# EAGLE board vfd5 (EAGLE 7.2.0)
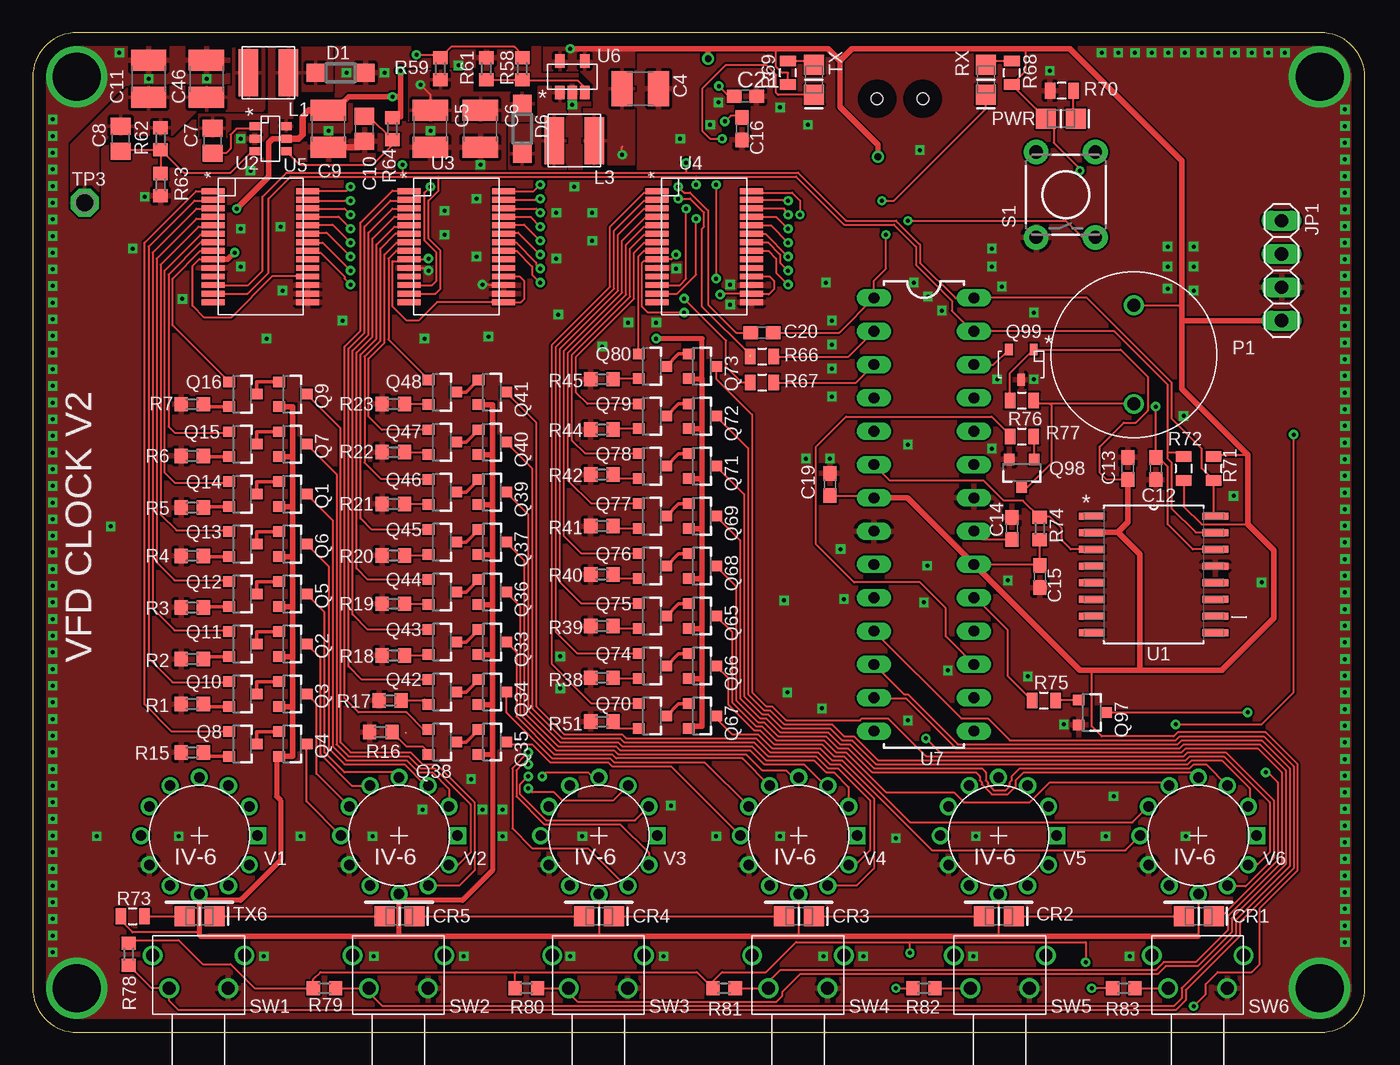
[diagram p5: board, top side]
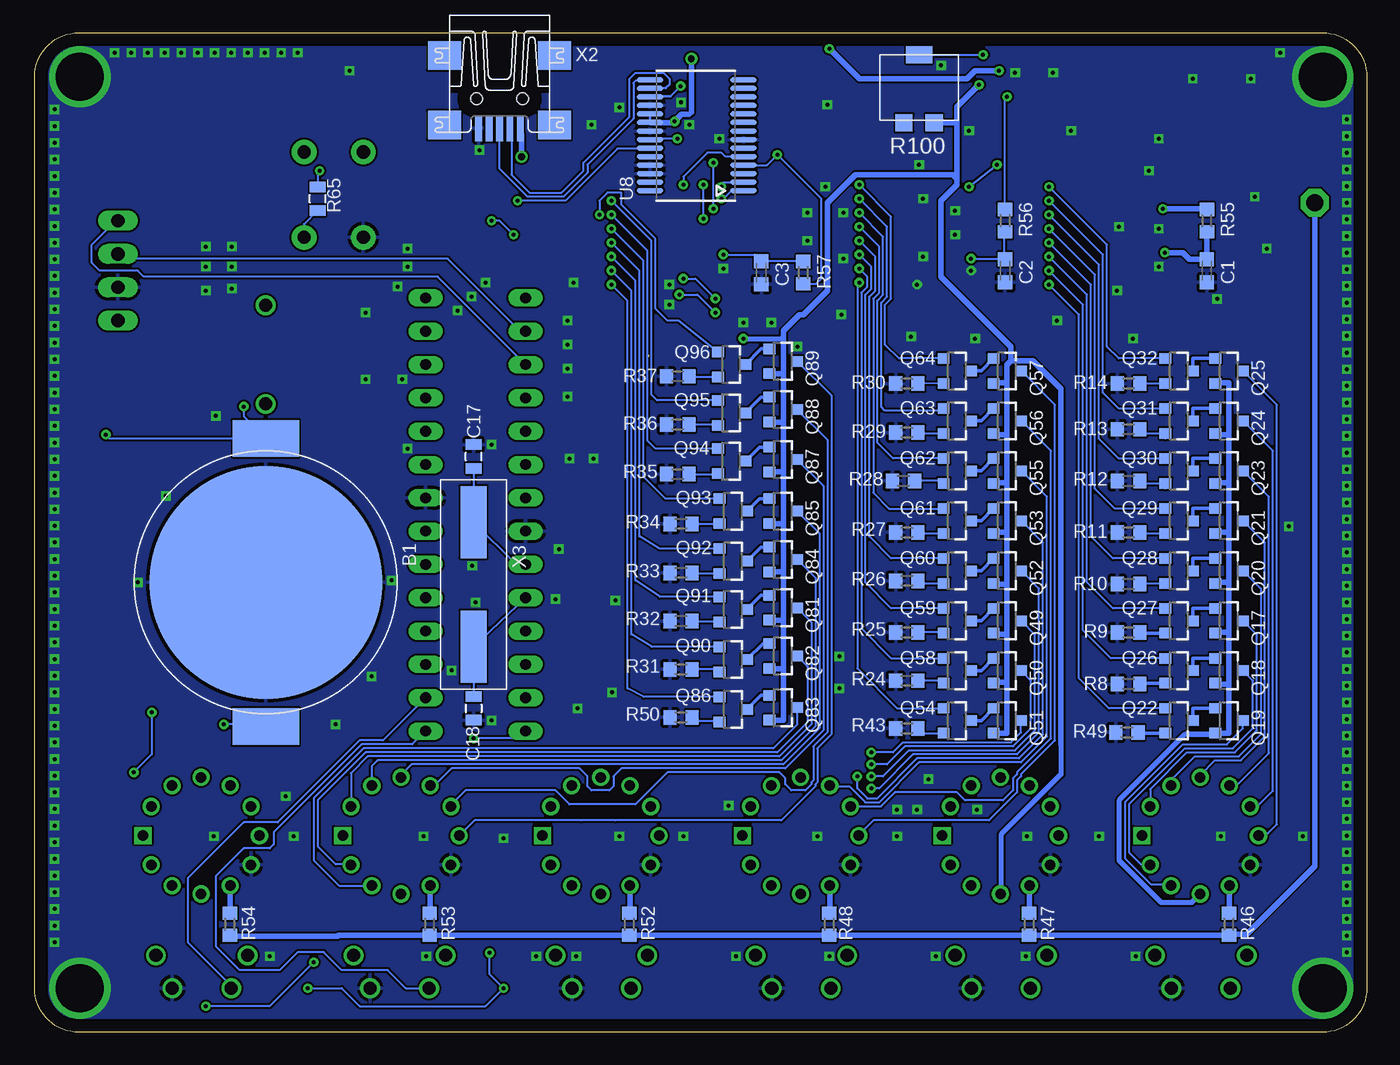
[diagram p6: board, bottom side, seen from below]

Size 101.6 x 76.2 mm. Coordinates in mm from the lower left corner, seen from the top.
Outline: 3.35,0 98.25,0 arc90 101.6,3.35 101.6,72.85 arc90 98.25,76.2 3.35,76.2 arc90 0,72.85 0,3.35 arc90 3.35,0
Copper layers (1*16): Top 0.035mm / dielectric 1.5mm / Bottom 0.035mm
Design rules "default *": minimum track width 6mil, minimum drill 12mil, track to track 6mil, track to pad 6mil, pad to pad 6mil, via to via 6mil, smd to smd 6mil, copper to edge 40mil, drill to drill 8mil, minimum pad ring 10mil, minimum via ring 8mil, stop-mask expansion 4mil, vias tented up to drill 12mil, thermal gap 10mil

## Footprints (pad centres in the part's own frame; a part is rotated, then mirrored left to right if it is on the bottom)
BK-912 = smd 2.79 x 5.08: +1 -10.985,0; +2 10.985,0 | smd 17.78 x 17.78: - 0,0
C0603K = smd 1.05 x 1.08: 1 -0.875,0; 2 0.875,0
C1210 = smd 1.6 x 2.7: 1 -1.4,0; 2 1.4,0
C0805 = smd 1.3 x 1.5: 1 -0.95,0; 2 0.95,0
C0603 = smd 1.1 x 1: 1 -0.85,0; 2 0.85,0
0805 = smd 0.8 x 1.2: 1 -0.9,0; 2 0.9,0
LED0805 = smd 1.524 x 1.524: 1 0,0; 2 2.286,0
SOD123 = smd 1.4 x 1.4: A 1.9,0; C -1.9,0
1X04 = drill 1.016 long: 1 -3.81,0; 2 -1.27,0; 3 1.27,0; 4 3.81,0
SRN4026 = smd 1.5 x 3.6: P$1 -1.525,0; P$2 1.525,0
PKM13EPYH4000-A0 = drill 1: P$1 0,3.76; P$2 0,-3.76
SOT23-3 = smd 0.8 x 0.9: 1 -0.95,-1; 2 0.95,-1; 3 0,1.1
SOT23-3' = smd 0.6 x 0.9: 1 0.32,-1.15; 2 2.22,-1.15; 3 1.27,1.15
R0603 = smd 1 x 1.1: 1 -0.85,0; 2 0.85,0
3224G = smd 1.3 x 1.3: 1 3.2,0.69; 3 3.2,-1.61 | smd 1.3 x 2: 2 -2,-0.46
TACTILE-PTH = drill 1.016 pad 1.88: 1 -3.251,2.261; 2 3.251,2.261; 3 -3.251,-2.261; 4 3.251,-2.261
EVQ-PF008K = drill 1: NC1 -3.5,2.5; NC2 3.5,2.5; S1 -2.25,0; S2 2.25,0
P1-13 = drill 1.321 pad 2.159 octagon: TP 0,0
SOIC127P1032X265-16N = smd 1.981 x 0.533: 1 -4.699,4.445; 2 -4.699,3.175; 3 -4.699,1.905; 4 -4.699,0.635; 5 -4.699,-0.635; 6 -4.699,-1.905; 7 -4.699,-3.175; 8 -4.699,-4.445; 9 4.699,-4.445; 10 4.699,-3.175; 11 4.699,-1.905; 12 4.699,-0.635; 13 4.699,0.635; 14 4.699,1.905; 15 4.699,3.175; 16 4.699,4.445
SSOP16 = smd 0.45 x 1.75: 1 -4.225,-3.6; 2 -3.575,-3.6; 3 -2.925,-3.6; 4 -2.275,-3.6; 5 -1.625,-3.6; 6 -0.975,-3.6; 7 -0.325,-3.6; 8 0.325,-3.6; 9 0.975,-3.6; 10 1.625,-3.6; 11 2.275,-3.6; 12 2.925,-3.6; 13 3.575,-3.6; 14 4.225,-3.6; 15 4.225,3.6; 16 3.575,3.6; 17 2.925,3.6; 18 2.275,3.6; 19 1.625,3.6; 20 0.975,3.6; 21 0.325,3.6; 22 -0.325,3.6; 23 -0.975,3.6; 24 -1.625,3.6; 25 -2.275,3.6; 26 -2.925,3.6; 27 -3.575,3.6; 28 -4.225,3.6
SOT236 = smd 0.63 x 0.8: 1 -0.95,-1.2; 2 0,-1.2; 3 0.95,-1.2; 4 0.95,1.2; 5 0,1.2; 6 -0.95,1.2
SOT23-5 = smd 0.7 x 1: 1 0.95,1.2; 2 0,1.2; 3 -0.95,1.2; 4 -0.95,-1.2; 5 0.95,-1.2
DIL28-3 = drill 0.813 long: 1 -16.51,-3.81; 2 -13.97,-3.81; 3 -11.43,-3.81; 4 -8.89,-3.81; 5 -6.35,-3.81; 6 -3.81,-3.81; 7 -1.27,-3.81; 8 1.27,-3.81; 9 3.81,-3.81; 10 6.35,-3.81; 11 8.89,-3.81; 12 11.43,-3.81; 13 13.97,-3.81; 14 16.51,-3.81; 15 16.51,3.81; 16 13.97,3.81; 17 11.43,3.81; 18 8.89,3.81; 19 6.35,3.81; 20 3.81,3.81; 21 1.27,3.81; 22 -1.27,3.81; 23 -3.81,3.81; 24 -6.35,3.81; 25 -8.89,3.81; 26 -11.43,3.81; 27 -13.97,3.81; 28 -16.51,3.81
SSOP28 = smd 0.381 x 2.032: 1 0,0; 2 0.65,0; 3 1.3,0; 4 1.95,0; 5 2.6,0; 6 3.25,0; 7 3.9,0; 8 4.55,0; 9 5.2,0; 10 5.85,0; 11 6.5,0; 12 7.15,0; 13 7.8,0; 14 8.45,0; 15 8.45,7.112; 16 7.8,7.112; 17 7.15,7.112; 18 6.5,7.112; 19 5.85,7.112; 20 5.2,7.112; 21 4.55,7.112; 22 3.9,7.112; 23 3.25,7.112; 24 2.6,7.112; 25 1.95,7.112; 26 1.3,7.112; 27 0.65,7.112; 28 0,7.112
IV6_NUMITRON_PAC = drill 0.8: BL -3.81,2.223; BOT -4.445,0; BR 2.223,-3.81; DOT 3.81,-2.223; FIL_M -3.81,-2.223; FIL_P -2.223,-3.81; GRID_P 0,-4.445; MID 0,4.445; TL -2.223,3.81; TOP 2.223,3.81; TR 3.81,2.223 | drill 0.8 square: NC 4.445,0
UX60-MB-5ST = smd 2 x 0.5: 1 2.25,1.6; 2 2.25,0.8; 3 2.25,0; 4 2.25,-0.8; 5 2.25,-1.6 | smd 2.2 x 2.5: M1 -3.3,-4.2; M2 -3.3,4.2; M3 2,4.2; M4 2,-4.2 | hole 0.9: 0,-1.75; 0,1.75
CSM7X = smd 5.5 x 2: P$1 4.75,0; P$2 -4.75,0

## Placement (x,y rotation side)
B1  BK-912  [BK-912]  83.97,34.29 270 bottom
C1  0.1uF  [C0603K]  12.19,58.06 270 bottom
C2  0.1uF  [C0603K]  27.58,58.06 270 bottom
C3  0.1uF  [C0603K]  46.18,57.91 270 bottom
C4  [C1210]  46.33,71.93 0 top
C5  10uF  [C1210]  30.33,68.88 270 top
C6  10uF  [C1210]  34.14,68.88 270 top
C7  0.1uF 25V  [C0805]  13.72,67.97 90 top
C8  DNI  [C0805]  6.71,68.12 90 top
C9  2.2uF 25V  [C1210]  22.56,68.88 270 top
C10  0.1uF 25V  [C0805]  25.3,68.88 270 top
C11  2.2uF 25V  [C1210]  8.84,72.69 90 top
C12  0.1uF  [C0603]  85.65,42.98 270 top
C13  0.1uF  [C0603]  83.52,42.98 90 top
C14  0.1uF  [C0603]  74.68,38.4 90 top
C15  0.1uF  [C0603]  76.81,34.75 270 top
C16  0.1uF  [C0603]  54.1,68.88 270 top
C17  22pf  [0805]  68.12,43.89 90 bottom
C18  22pf  [0805]  68.12,24.69 270 bottom
C19  [C0603]  60.81,41.76 90 top
C20  0.1uF  [C0603]  55.63,53.34 180 top
C21  0.1uF  [C0603]  54.36,71.37 0 top
C46  22uF 10V Tant.  [C1210]  13.26,72.69 90 top
CR1  GREEN_TX  [LED0805]  90.07,8.84 180 top
CR2  GREEN_TX  [LED0805]  74.83,8.84 180 top
CR3  GREEN_TX  [LED0805]  59.59,8.84 180 top
CR4  GREEN_TX  [LED0805]  44.35,8.84 180 top
CR5  GREEN_TX  [LED0805]  29.11,8.84 180 top
D1  RF081M2SCT-ND  [SOD123]  23.47,73.15 0 top
D6  RF081M2SCT-ND  [SOD123]  37.34,68.88 270 top
JP1  [1X04]  95.25,58.06 270 top
L1  SRN4026-303M  [SRN4026]  17.98,73.15 180 top
L3  SRN4026-303M  [SRN4026]  41.3,67.97 180 top
P1  PKM13EPYH4000-A0  [PKM13EPYH4000-A0]  83.97,51.66 0 top
PWR  PWR  [LED0805]  79.55,69.65 180 top
Q1  [SOT23-3]  19.79,41.02 270 top
Q2  [SOT23-3]  19.79,29.59 270 top
Q3  [SOT23-3]  19.79,25.78 270 top
Q4  [SOT23-3]  19.79,21.97 270 top
Q5  [SOT23-3]  19.79,33.4 270 top
Q6  [SOT23-3]  19.79,37.21 270 top
Q7  [SOT23-3]  19.79,44.83 270 top
Q8  [SOT23-3]  15.98,21.97 270 top
Q9  [SOT23-3]  19.79,48.64 270 top
Q10  [SOT23-3]  15.98,25.78 270 top
Q11  [SOT23-3]  15.98,29.59 270 top
Q12  [SOT23-3]  15.98,33.4 270 top
Q13  [SOT23-3]  15.98,37.21 270 top
Q14  [SOT23-3]  15.98,41.02 270 top
Q15  [SOT23-3]  15.98,44.83 270 top
Q16  [SOT23-3]  15.98,48.64 270 top
Q17  [SOT23-3]  10.54,31.37 270 bottom
Q18  [SOT23-3]  10.54,27.56 270 bottom
Q19  [SOT23-3]  10.54,23.75 270 bottom
Q20  [SOT23-3]  10.54,35.18 270 bottom
Q21  [SOT23-3]  10.54,38.99 270 bottom
Q22  [SOT23-3]  14.35,23.75 270 bottom
Q23  [SOT23-3]  10.54,42.8 270 bottom
Q24  [SOT23-3]  10.54,46.61 270 bottom
Q25  [SOT23-3]  10.54,50.42 270 bottom
Q26  [SOT23-3]  14.35,27.56 270 bottom
Q27  [SOT23-3]  14.35,31.37 270 bottom
Q28  [SOT23-3]  14.35,35.18 270 bottom
Q29  [SOT23-3]  14.35,38.99 270 bottom
Q30  [SOT23-3]  14.35,42.8 270 bottom
Q31  [SOT23-3]  14.35,46.61 270 bottom
Q32  [SOT23-3]  14.35,50.42 270 bottom
Q33  [SOT23-3]  35,29.74 270 top
Q34  [SOT23-3]  35,25.93 270 top
Q35  [SOT23-3]  35,22.12 270 top
Q36  [SOT23-3]  35,33.55 270 top
Q37  [SOT23-3]  35,37.36 270 top
Q38  [SOT23-3]  31.19,22.12 270 top
Q39  [SOT23-3]  35,41.17 270 top
Q40  [SOT23-3]  35,44.98 270 top
Q41  [SOT23-3]  35,48.79 270 top
Q42  [SOT23-3]  31.19,25.93 270 top
Q43  [SOT23-3]  31.19,29.74 270 top
Q44  [SOT23-3]  31.19,33.55 270 top
Q45  [SOT23-3]  31.19,37.36 270 top
Q46  [SOT23-3]  31.19,41.17 270 top
Q47  [SOT23-3]  31.19,44.98 270 top
Q48  [SOT23-3]  31.19,48.79 270 top
Q49  [SOT23-3]  27.46,31.37 270 bottom
Q50  [SOT23-3]  27.46,27.56 270 bottom
Q51  [SOT23-3]  27.46,23.75 270 bottom
Q52  [SOT23-3]  27.46,35.18 270 bottom
Q53  [SOT23-3]  27.46,38.99 270 bottom
Q54  [SOT23-3]  31.27,23.75 270 bottom
Q55  [SOT23-3]  27.46,42.8 270 bottom
Q56  [SOT23-3]  27.46,46.61 270 bottom
Q57  [SOT23-3]  27.46,50.42 270 bottom
Q58  [SOT23-3]  31.27,27.56 270 bottom
Q59  [SOT23-3]  31.27,31.37 270 bottom
Q60  [SOT23-3]  31.27,35.18 270 bottom
Q61  [SOT23-3]  31.27,38.99 270 bottom
Q62  [SOT23-3]  31.27,42.8 270 bottom
Q63  [SOT23-3]  31.27,46.61 270 bottom
Q64  [SOT23-3]  31.27,50.42 270 bottom
Q65  [SOT23-3]  51.03,31.72 270 top
Q66  [SOT23-3]  51.03,27.91 270 top
Q67  [SOT23-3]  51.03,24.1 270 top
Q68  [SOT23-3]  51.03,35.53 270 top
Q69  [SOT23-3]  51.03,39.34 270 top
Q70  [SOT23-3]  47.22,24.1 270 top
Q71  [SOT23-3]  51.03,43.15 270 top
Q72  [SOT23-3]  51.03,46.96 270 top
Q73  [SOT23-3]  51.03,50.77 270 top
Q74  [SOT23-3]  47.22,27.91 270 top
Q75  [SOT23-3]  47.22,31.72 270 top
Q76  [SOT23-3]  47.22,35.53 270 top
Q77  [SOT23-3]  47.22,39.34 270 top
Q78  [SOT23-3]  47.22,43.15 270 top
Q79  [SOT23-3]  47.22,46.96 270 top
Q80  [SOT23-3]  47.22,50.77 270 top
Q81  [SOT23-3]  44.55,32.36 270 bottom
Q82  [SOT23-3]  44.55,28.68 270 bottom
Q83  [SOT23-3]  44.55,24.74 270 bottom
Q84  [SOT23-3]  44.55,36.04 270 bottom
Q85  [SOT23-3]  44.55,39.73 270 bottom
Q86  [SOT23-3]  48.36,24.61 270 bottom
Q87  [SOT23-3]  44.55,43.66 270 bottom
Q88  [SOT23-3]  44.55,47.47 270 bottom
Q89  [SOT23-3]  44.55,51.16 270 bottom
Q90  [SOT23-3]  48.36,28.42 270 bottom
Q91  [SOT23-3]  48.36,32.23 270 bottom
Q92  [SOT23-3]  48.36,35.92 270 bottom
Q93  [SOT23-3]  48.36,39.73 270 bottom
Q94  [SOT23-3]  48.49,43.54 270 bottom
Q95  [SOT23-3]  48.49,47.22 270 bottom
Q96  [SOT23-3]  48.49,50.9 270 bottom
Q97  [SOT23-3]  80.77,24.38 270 top
Q98  [SOT23-3]  75.44,42.67 180 top
Q99  MCP9700  [SOT23-3']  76.66,50.9 180 top
R1  10k  [R0603]  12.17,25.02 0 top
R2  10k  [R0603]  12.17,28.45 0 top
R3  10k  [R0603]  12.17,32.38 0 top
R4  10k  [R0603]  12.17,36.32 0 top
R5  10k  [R0603]  12.17,40.01 0 top
R6  10k  [R0603]  12.17,43.94 0 top
R7  10k  [R0603]  12.17,47.88 0 top
R8  10k  [R0603]  18.16,26.54 0 bottom
R9  10k  [R0603]  18.16,30.48 0 bottom
R10  10k  [R0603]  18.16,34.16 0 bottom
R11  10k  [R0603]  18.16,38.1 0 bottom
R12  10k  [R0603]  18.16,42.04 0 bottom
R13  10k  [R0603]  18.16,45.97 0 bottom
R14  10k  [R0603]  18.16,49.45 0 bottom
R15  10k  [R0603]  12.17,21.34 0 top
R16  10k  [R0603]  26.54,22.89 0 top
R17  10k  [R0603]  27.25,25.3 0 top
R18  10k  [R0603]  27.51,28.73 0 top
R19  10k  [R0603]  27.51,32.66 0 top
R20  10k  [R0603]  27.51,36.35 0 top
R21  10k  [R0603]  27.51,40.28 0 top
R22  10k  [R0603]  27.51,44.22 0 top
R23  10k  [R0603]  27.51,47.9 0 top
R24  10k  [R0603]  35.08,26.8 0 bottom
R25  10k  [R0603]  35.08,30.48 0 bottom
R26  10k  [R0603]  35.08,34.42 0 bottom
R27  10k  [R0603]  35.08,38.1 0 bottom
R28  10k  [R0603]  35.33,42.04 0 bottom
R29  10k  [R0603]  35.08,45.72 0 bottom
R30  10k  [R0603]  35.08,49.45 0 bottom
R31  10k  [R0603]  52.3,27.66 0 bottom
R32  10k  [R0603]  52.3,31.34 0 bottom
R33  10k  [R0603]  52.3,35.03 0 bottom
R34  10k  [R0603]  52.3,38.76 0 bottom
R35  10k  [R0603]  52.55,42.55 0 bottom
R36  10k  [R0603]  52.55,46.33 0 bottom
R37  10k  [R0603]  52.55,50.01 0 bottom
R38  10k  [R0603]  43.41,27.03 0 top
R39  10k  [R0603]  43.41,30.96 0 top
R40  10k  [R0603]  43.41,34.9 0 top
R41  10k  [R0603]  43.41,38.58 0 top
R42  10k  [R0603]  43.41,42.52 0 top
R43  10k  [R0603]  35.08,23.16 0 bottom
R44  10k  [R0603]  43.41,45.95 0 top
R45  10k  [R0603]  43.41,49.78 0 top
R46  [R0603]  10.52,8.23 270 bottom
R47  10  [R0603]  25.76,8.23 270 bottom
R48  10  [R0603]  41,8.23 270 bottom
R49  10k  [R0603]  18.29,22.86 0 bottom
R50  10k  [R0603]  52.3,24 0 bottom
R51  10k  [R0603]  43.41,23.67 0 top
R52  10  [R0603]  56.24,8.23 270 bottom
R53  10  [R0603]  71.48,8.23 270 bottom
R54  10  [R0603]  86.72,8.23 270 bottom
R55  10  [R0603]  12.19,61.87 270 bottom
R56  10  [R0603]  27.58,61.87 270 bottom
R57  10  [R0603]  42.98,57.91 90 bottom
R58  10k  [R0603]  37.34,73.46 90 top
R59  100k  [R0603]  31.09,73.46 270 top
R61  3k  [R0603]  34.59,73.46 270 top
R62  49.9k  [R0603]  9.75,68.12 90 top
R63  15.8k  [R0603]  9.75,64.62 90 top
R64  49.9k  [R0603]  27.43,68.88 90 top
R65  10k  [0805]  80.01,63.55 90 bottom
R66  1k  [0805]  55.63,51.51 0 top
R67  1k  [0805]  55.63,49.53 0 top
R68  330  [0805]  74.68,73.15 90 top
R69  330  [0805]  57.61,73.15 90 top
R70  330  [0805]  78.49,71.78 180 top
R71  2.2k  [0805]  90.07,42.98 90 top
R72  2.2k  [0805]  87.78,42.98 270 top
R73  1k  [0805]  7.62,8.84 0 top
R74  1k  [R0603]  76.81,38.4 90 top
R75  1k  [0805]  77.11,25.3 0 top
R76  1k  [0805]  75.44,48.16 0 top
R77  1k  [0805]  75.44,45.42 0 top
R78  1k  [R0603]  7.32,5.94 270 top
R79  1k  [R0603]  22.25,3.35 0 top
R80  1k  [R0603]  37.64,3.35 0 top
R81  1k  [R0603]  52.73,3.35 0 top
R82  1k  [R0603]  67.97,3.35 0 top
R83  1k  [R0603]  83.21,3.35 0 top
R100  3224G-1-104E  [3224G]  33.68,72.54 270 bottom
RX  RED_RX  [LED0805]  72.69,71.48 90 top
S1  SWITCH-MOMENTARY-2PTH  [TACTILE-PTH]  78.79,63.86 90 top
SW1  EVQ-PF008K  [EVQ-PF008K]  12.65,3.35 0 top
SW2  EVQ-PF008K  [EVQ-PF008K]  27.89,3.35 0 top
SW3  EVQ-PF008K  [EVQ-PF008K]  43.13,3.35 0 top
SW4  EVQ-PF008K  [EVQ-PF008K]  58.37,3.35 0 top
SW5  EVQ-PF008K  [EVQ-PF008K]  73.76,3.35 0 top
SW6  EVQ-PF008K  [EVQ-PF008K]  88.85,3.35 0 top
TP3  TPPAD1-13  [P1-13]  3.96,63.25 0 top
TX  GREEN_TX  [LED0805]  59.59,71.48 90 top
TX6  GREEN_TX  [LED0805]  13.87,8.84 180 top
U1  DS3231S  [SOIC127P1032X265-16N]  85.5,34.9 0 top
U2  MCP23017  [SSOP16]  17.37,59.89 270 top
U3  MCP23017  [SSOP16]  32.31,59.89 270 top
U4  MCP23017  [SSOP16]  51.21,59.89 270 top
U5  AOZ128CI-1  [SOT236]  18.14,68.12 270 top
U6  MIC2288  [SOT23-5]  41.15,72.85 180 top
U7  ATMEGA328P_PDIP  [DIL28-3]  67.97,39.47 270 top
U8  FT232RL  [SSOP28]  47.55,64.16 90 bottom
V1  IV6_NUMITRON  [IV6_NUMITRON_PAC]  12.7,14.99 0 top
V2  IV6_NUMITRON  [IV6_NUMITRON_PAC]  27.94,14.99 0 top
V3  IV6_NUMITRON  [IV6_NUMITRON_PAC]  43.18,14.99 0 top
V4  IV6_NUMITRON  [IV6_NUMITRON_PAC]  58.42,14.99 0 top
V5  IV6_NUMITRON  [IV6_NUMITRON_PAC]  73.66,14.99 0 top
V6  IV6_NUMITRON  [IV6_NUMITRON_PAC]  88.9,14.99 0 top
X2  MINI-USB-UX60-MB-5ST  [UX60-MB-5ST]  66.14,71.17 270 bottom
X3  ECS-80-20  [CSM7X]  68.12,34.14 270 bottom

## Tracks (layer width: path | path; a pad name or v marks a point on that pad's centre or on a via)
+5V  (via drill 0.3, 0.51)
  Top 0.152: 55.93,74.83 56.08,74.98 | 75.74,74.98 75.74,73.32 R68.1 74.68,72.24 PWR.2 77.88,69.04 77.88,67.82 79.86,65.84 v79.86,65.68 | R69.1 57.61,73.15 57.15,73.15 56.69,73.61 56.69,74.83 56.54,74.98 | v44.96,66.9 44.96,67.51 | U7.20 76.75,35.66 C15.1 R74.1 | C19.1 63.99,40.91 U7.7 | R71.2 90.23,44.04 92.66,44.04 | R72.2 87.78,40.08 89.15,38.71 92.66,38.71 | C16.1 53.94,69.88 53.24,69.88 v52.78,69.44 | R76.1 74.54,50.25 Q99.1 82.97,52.05 85.04,49.99 85.04,47.4 84.12,46.48 83.21,46.48 81.38,44.65 81.38,42.67 81.93,42.13 C13.1 | P1.P$1 87.38,55.42 87.63,55.17 | R78.1 7.32,6.86 7.47,7.01 11.12,7.01 12.95,5.18 15.09,5.18 16.92,3.35 R79.1 21.4,4.03 21.95,4.57 36.88,4.57 | 36.88,4.57 50.66,4.57 R81.1 51.88,3.87 52.58,4.57 55.93,4.57 58.22,6.86 66.9,6.86 | R80.1 36.79,4.48 36.88,4.57 | v65.84,3.35 R82.1 | R83.1 v80.77,3.35 | 66.9,6.86 80.31,6.86 v80.31,5.33 | v66.9,6.04 66.9,6.86 | v88.54,1.98 89.46,2.9 89.46,3.66 90.37,4.57 92.96,4.57 93.57,5.18 93.57,9.45 96.47,12.34 96.47,20.42 94.03,22.86 87.33,22.86 87.02,22.55 81.53,22.55 80.77,23.32 80.77,27.58
  Top 0.406: v64.47,66.75 64.47,67.67 61.57,70.56 61.57,74.07 | 51.51,74.98 56.08,74.98 56.54,74.98 60.66,74.98 61.57,74.07 | 51.51,74.98 v41,74.98 | 40.2,74.18 U6.5 | U6.4 42.22,74.16 | v51.51,74.22 51.51,74.98 | 61.57,74.07 62.48,74.98 75.74,74.98 79.1,74.98 87.63,66.45 87.63,55.17 87.63,54.25 | v28.04,73.3 28.04,71.48 | 28.04,71.48 28.04,69.8 27.43,69.8 R64.2 | C9.1 23.04,70.28 24.08,71.32 v27.43,71.32 27.89,71.32 28.04,71.48 | U5.5 18.29,68.12 17.98,67.82 17.98,65.23 v15.54,62.79 | 84.43,27.58 90.68,27.58 94.64,31.55 94.64,36.73 92.66,38.71 92.66,44.04 87.63,49.07 87.63,54.25 | 84.43,27.58 80.77,27.58 79.86,27.58 U7.20 66.7,40.74 U7.7 | U1.2 80.82,38.1 82.75,38.1 | 82.75,38.1 84.43,36.42 84.43,27.58 | C13.1 83.52,38.86 82.75,38.1 | 87.63,54.25 JP1.4
  Top 0.508: U5.5 20.27,68.12 20.57,68.43 20.57,69.8 21.06,70.28 C9.1
  Bottom 0.152: v79.86,65.68 80.01,65.53 R65.2 | R56.1 27.58,71.17 v27.43,71.32 | U8.4 45.75,66.11 v44.96,66.9 41.6,63.55 41.6,57.45 42,57.06 R57.1 | v80.77,3.35 78.18,3.35 76.81,1.98 67.21,1.98 v65.84,3.35 66.9,4.42 v66.9,6.04 | v80.31,5.33 83.67,1.98 v88.54,1.98
  Bottom 0.203: U8.19 U8.20
  Bottom 0.406: X2.1 64.47,68.39 v64.47,66.75 | U8.20 54.64,69.34 52.88,69.34 v52.78,69.44 52.25,69.98 51.69,69.98 51.51,70.16 v51.51,74.22 | v15.54,62.79 12.26,62.79 R55.1 | v41,74.98 38.71,72.69 30.48,72.69 29.87,73.3 v28.04,73.3
  pour Top: 39.47,75.13 45.87,75.13 45.87,66.14 42.06,66.14 42.06,70.41 42.82,70.41 42.82,72.24 41.76,73.3 39.01,73.3 39.01,75.13
ALARM
  Top 0.152: U7.17 69.65,30.18 69.65,32.31 67.67,34.29 62.64,34.29 59.74,37.19 59.74,44.65 62.03,46.94 73.15,46.94 74.54,45.55 R77.1
FIL
  Bottom 0.406: R54.2 86.65,7.32 78.49,7.32 78.42,7.38 R53.2 R52.2 R48.2 R47.2 R46.2 10.43,7.47 9.14,7.47 3.96,12.65 TP3.TP
  pour Top: 17.53,74.98 15.24,74.98 15.24,72.09 7.32,72.09 2.9,67.67 2.9,62.79 5.03,62.79 5.03,67.51 5.94,68.43 10.67,68.43 12.5,70.26 17.53,70.26 17.68,70.41 17.68,74.98
GND  (via drill 0.3, 3.66)
  Top 0.152: U3.17 34.78,56.97 34.75,57 v34.29,57 | U3.10 29.97,58.27 v30.18,58.06
  Top 0.508: C10.2 24.85,67.48 C9.2
  Bottom 0.152: v30.18,58.06 30.48,58.06 | v34.29,57 34.29,57.3 | 83.36,34.9 B1.- 84.58,34.9
  other vias: 3.35,3.35 98.15,3.35 98.15,72.85 3.35,72.85 23.93,73.15 26.82,73.15 8.53,63.7 15.85,68.12 22.56,68.73 30.33,68.73 34.14,66.14 41.15,70.71 8.84,72.69 13.26,72.69 49.07,58.22 53.19,57 53.19,55.47 67.67,67.26 57,70.51 32.46,73.71 11.4,55.91 15.85,58.37 51.66,69.19 66.75,44.81 66.75,23.77 78.64,23.47 40.23,28.65 40.23,26.21 15.85,61.26 16.61,65.68 18.9,61.42 19.05,56.54 23.62,54.25 29.87,52.88 31.39,62.64 31.39,60.81 33.83,63.55 33.83,59.13 39.93,62.48 39.93,58.98 42.67,62.48 42.67,60.35 34.75,53.04 40.08,54.71 45.42,54.1 43.43,52.27 47.55,54.1 41.3,64.47 49.38,68.12 59.13,69.19 77.57,73.3 76.35,54.86 60.5,57.15 60.81,43.74 57.3,32.92 11.13,14.94 25.91,14.94 20.42,14.94 4.88,14.94 35.81,14.94 41.91,14.94 52.12,14.94 57,14.94 65.84,14.78 71.93,14.94 81.84,14.94 87.93,14.94 82.45,17.98 75.9,27.13 69.8,27.58 60.2,24.69 7.62,59.74 5.94,38.56 17.83,52.88 67.21,57.15 73.15,59.74 73.15,58.37 68.28,56.08 69.34,55.02 60.96,54.25 60.96,52.43 60.96,50.6 60.96,48.46 73.15,44.5 58.98,43.74 74.37,34.44 93.73,34.29 73.91,56.85 86.56,59.89 86.56,58.37 86.56,56.69 88.54,56.54 88.54,58.37 88.54,59.89 1.52,6.1 1.52,7.37 1.52,8.64 1.52,9.91 1.52,11.18 1.52,12.45 1.52,13.72 1.52,14.99 1.52,16.26 1.52,17.53 1.52,18.8 1.52,20.07 1.52,21.34 1.52,22.61 1.52,23.88 1.52,25.15 1.52,26.42 1.52,27.69 1.52,28.96 1.52,30.23 1.52,31.5 1.52,32.77 1.52,34.04 1.52,35.31 1.52,36.58 1.52,37.85 1.52,39.12 1.52,40.39 1.52,41.66 1.52,42.93 1.52,44.2 1.52,45.47 1.52,46.74 1.52,48.01 1.52,49.28 1.52,50.55 1.52,51.82 1.52,53.09 1.52,54.36 1.52,55.63 1.52,56.9 1.52,58.17 1.52,59.44 1.52,60.71 1.52,61.98 1.52,63.25 1.52,64.52 1.52,65.79 1.52,67.06 1.52,68.33 1.52,69.6 6.6,74.68 81.53,74.68 82.8,74.68 84.07,74.68 85.34,74.68 86.61,74.68 87.88,74.68 89.15,74.68 91.69,74.68 90.42,74.68 92.96,74.68 94.23,74.68 95.5,74.68 100.08,70.36 100.08,69.09 100.08,67.82 100.08,66.55 100.08,65.28 100.08,64.01 100.08,62.74 100.08,61.47 100.08,60.2 100.08,58.93 100.08,57.66 100.08,56.39 100.08,55.12 100.08,53.85 100.08,52.58 100.08,51.31 100.08,50.04 100.08,48.77 100.08,47.5 100.08,46.23 100.08,44.96 100.08,43.69 100.08,42.42 100.08,41.15 100.08,39.88 100.08,38.61 100.08,37.34 100.08,36.07 100.08,34.8 100.08,33.53 100.08,32.26 100.08,30.99 100.08,29.72 100.08,28.45 100.08,27.18 100.08,25.91 100.08,24.64 100.08,23.37 100.08,22.1 100.08,20.83 100.08,19.56 100.08,18.29 100.08,17.02 100.08,15.75 100.08,14.48 100.08,13.21 100.08,11.94 100.08,10.67 100.08,9.4 100.08,8.13 100.08,6.86 76.35,49.78 73.56,49.78 87.78,46.99 91.59,40.89 68.22,35.56 67.97,32.77 61.87,33.02 61.62,36.83 57.56,25.91 48.67,17.27 33.43,19.3 35.81,16.97 34.29,16.97 29.72,16.97 17.63,5.79 26.01,5.79 32.87,5.79 41,5.79 48.11,5.79 60.3,5.79 63.35,5.79 71.73,5.79 83.67,5.79 52.3,70.89
  pour Top (rank 5): 0,80.01 101.35,79.76 100.33,0 0,0
  pour Bottom: 0.51,79.12 112.37,78.97 112.37,3.71 arc-90 109.01,0.36 0.51,0.51
INTERUPT
  Top 0.152: U1.3 79.17,36.8 78.49,37.49 78.49,38.41 77.57,39.32 76.87,39.32 R74.2 75.53,40.54 74.07,40.54 72.54,42.06 65.38,42.06 U7.6
LIGHT
  Top 0.152: R75.1 74.37,27.14 74.37,30.63 71.88,33.12 U7.19
N$1
  Top 0.152: 36.27,21.95 38.09,21.95 39.47,20.57 43.89,20.57 44.2,20.27 48.69,20.27 V4.BOT
  Top 0.254: Q35.3 36.27,21.95
N$2  (via drill 0.3)
  Top 0.152: U2.21 21.11,59.44 21.95,59.44 23.77,57.61 23.77,57.45 v24.23,57
  Bottom 0.152: Q22.1 15.36,24.69 19.66,24.69 21.95,26.98 21.95,54.71 v24.23,57
N$3
  Bottom 0.152: Q17.3 8.38,30.31 8.38,23.01 10.06,21.34 13.72,21.34 16.51,18.54 V1.TR
N$4
  Top 0.152: 20.89,21.65 Q4.3 20.89,17.59 V2.BOT
N$5
  Bottom 0.152: R14.2 17.3,49.47 Q32.2
N$6
  Top 0.152: Q3.3 21.64,25.03 21.64,19.7 V2.BL
N$7
  Top 0.152: Q2.3 21.95,28.53 21.95,21.18 24.33,18.8 V2.TL
N$8
  Top 0.152: Q5.3 22.25,32.04 22.25,21.34 23.77,19.81 27.56,19.81 V2.MID
N$9
  Top 0.152: Q6.3 22.55,35.54 22.55,21.64 23.77,20.42 28.35,20.42 29.97,18.8 V2.TOP 30.12,18.8
N$10
  Top 0.152: Q1.3 22.86,39.05 22.86,21.79 23.93,20.73 28.5,20.73 29.41,19.81 30.48,19.81 31.75,18.54 V2.TR
N$11
  Top 0.152: Q7.3 23.16,42.55 23.16,21.95 24.08,21.03 28.65,21.03 29.57,20.12 30.63,20.12 33.38,17.37 33.38,13.72 32.42,12.76 V2.DOT
N$12  (via drill 0.3)
  Top 0.152: U2.22 20.99,60.2 22.1,60.2 v24.23,58.06
  Bottom 0.152: Q26.1 15.36,28.5 19.51,28.5 21.64,30.63 21.64,55.47 v24.23,58.06
N$13
  Top 0.152: Q9.3 23.47,46.06 23.47,22.1 24.23,21.34 28.8,21.34 29.72,20.42 30.79,20.42 33.68,17.53 33.68,12.34 32.51,11.18 V2.BR
N$14
  Top 0.254: Q8.3 17.08,22.92 Q4.1
N$15
  Top 0.254: Q10.3 17.08,26.73 Q3.1
N$16
  Top 0.254: Q11.3 17.08,30.54 Q2.1
N$17
  Top 0.254: Q12.3 17.08,34.35 Q5.1
N$18
  Top 0.254: Q13.3 17.08,38.16 Q6.1
N$19
  Top 0.254: Q14.3 17.08,41.97 Q1.1
N$20
  Top 0.254: Q15.3 17.08,45.78 Q7.1
N$21
  Bottom 0.152: Q18.3 8.69,26.8 8.69,23.16 10.21,21.64 13.87,21.64 18.14,17.37 18.14,13.72 17.22,12.8 16.55,12.8 V1.DOT
N$22
  Top 0.254: Q16.3 17.08,49.59 Q9.1
N$23
  Top 0.254: 13.12,28.64 Q11.2
  Top 0.406: 13.12,28.64 13.02,28.64 R2.2
N$24
  Top 0.254: 13.12,32.45 Q12.2
  Top 0.406: R3.2 13.12,32.38 13.12,32.45
N$25
  Top 0.254: 13.12,21.02 Q8.2
  Top 0.406: 13.12,21.02 13.02,21.02 R15.2
N$26
  Top 0.254: 13.12,36.26 Q13.2
  Top 0.406: 13.12,36.26 13.02,36.26 R4.2
N$27
  Top 0.254: Q16.2 13.02,47.69 R7.2
N$28
  Top 0.254: 14.98,40.39 Q14.2 13.02,40.07 R5.2
N$29
  Top 0.254: 14.98,44.2 Q15.2 13.02,43.88 R6.2
N$30
  Top 0.254: 13.12,24.83 Q10.2
  Top 0.406: R1.2 13.12,25.02 13.12,24.83
N$31
  Top 0.152: Q8.1 10.61,22.92 8.53,24.99 8.53,60.2 12.46,64.12 U2.1
N$32
  Top 0.152: Q10.1 14.92,26.67 10.67,26.67 8.84,28.5 8.84,59.89 12.34,63.4 13.7,63.4 U2.2
N$33
  Top 0.152: Q11.1 14.88,30.63 10.82,30.63 9.14,32.31 9.14,59.44 12.5,62.79 13.74,62.79 U2.3
N$34
  Top 0.152: Q12.1 14.88,34.44 10.82,34.44 9.45,35.81 9.45,58.98 12.5,62.03 13.63,62.03 U2.4
N$35
  Top 0.152: Q13.1 14.88,38.25 10.97,38.25 9.75,39.47 9.75,58.52 12.65,61.42 13.67,61.42 U2.5
N$36
  Top 0.152: Q14.1 14.92,41.91 10.82,41.91 10.06,42.67 10.06,58.06 12.8,60.81 13.71,60.81 U2.6
N$37
  Top 0.152: Q15.1 14.92,45.72 10.82,45.72 10.36,46.18 10.36,57.76 12.82,60.22 U2.7
N$38
  Top 0.152: Q16.1 10.67,53.9 10.67,57.45 12.78,59.57 U2.8
N$39
  Bottom 0.152: Q21.3 7.77,37.32 7.77,22.55 9.6,20.73 11.58,20.73 12.7,19.61 V1.MID
N$40
  Bottom 0.152: Q23.3 7.47,40.83 7.47,21.27 9.94,18.8 V1.TL
N$41
  Bottom 0.152: Q24.3 7.16,44.33 7.16,18.4 8.36,17.21 V1.BL
N$42
  Bottom 0.152: Q25.3 6.86,47.84 6.86,15.85 7.72,14.99 V1.BOT
N$43
  Bottom 0.254: Q19.1 13.25,24.7 Q22.3
N$44
  Bottom 0.254: Q18.1 13.25,28.51 Q26.3
N$45
  Bottom 0.254: Q17.1 13.25,32.32 Q27.3
N$46
  Bottom 0.254: Q20.1 13.25,36.13 Q28.3
N$47
  Bottom 0.254: Q21.1 13.25,39.94 Q29.3
N$48
  Bottom 0.254: Q23.1 13.25,43.75 Q30.3
N$49
  Bottom 0.254: Q24.1 13.25,47.56 Q31.3
N$50
  Bottom 0.254: Q25.1 13.25,51.37 Q32.3
N$51
  Bottom 0.152: Q64.2 33.96,49.45 R30.2
N$52
  Bottom 0.152: R9.2 17.25,30.42 Q27.2
  Bottom 0.254: Q27.2 17.21,30.42
N$53
  Bottom 0.152: R10.2 17.25,34.23 Q28.2
  Bottom 0.254: 15.35,33.91 Q28.2
N$54
  Bottom 0.152: R11.2 17.25,38.04 Q29.2
  Bottom 0.254: 15.35,37.72 Q29.2
N$55
  Bottom 0.152: R12.2 17.12,41.85 Q30.2
  Bottom 0.254: 15.35,41.53 Q30.2
N$56
  Top 0.152: R23.2 30.13,47.9 Q48.2
N$57
  Bottom 0.406: V2.FIL_P 25.72,9.12 R47.1
N$58
  Bottom 0.152: R13.2 17,45.66 Q31.2
  Bottom 0.254: 15.35,45.34 Q31.2
N$59
  Bottom 0.152: R8.2 17.25,26.61 17.21,26.61
  Bottom 0.254: Q26.2 17.21,26.61
N$60  (via drill 0.3)
  Top 0.152: U2.23 21.07,60.96 22.4,60.96 v24.23,59.13
  Bottom 0.152: Q27.1 15.36,32.31 19.36,32.31 21.34,34.29 21.34,56.24 v24.23,59.13
N$61  (via drill 0.3)
  Top 0.152: U2.24 21.02,61.57 22.86,61.57 v24.23,60.2
  Bottom 0.152: Q28.1 15.36,36.12 19.36,36.12 21.03,37.8 21.03,57 v24.23,60.2
N$62  (via drill 0.3)
  Top 0.152: U2.25 20.98,62.18 23.32,62.18 v24.23,61.27
  Bottom 0.152: Q29.1 15.36,39.93 19.2,39.93 20.73,41.45 20.73,57.76 v24.23,61.27
N$63  (via drill 0.3)
  Top 0.152: U2.26 21,62.79 23.77,62.79 v24.23,62.33
  Bottom 0.152: Q30.1 15.36,43.74 18.9,43.74 20.42,45.26 20.42,58.52 v24.23,62.33
N$64  (via drill 0.3)
  Top 0.152: U2.27 21.04,63.4 v24.23,63.4
  Bottom 0.152: Q31.1 15.36,47.55 18.9,47.55 20.12,48.77 20.12,59.28 v24.23,63.4
N$65  (via drill 0.3)
  Top 0.152: 21.02,64.16 U2.28 23.89,64.12 v24.23,64.47
  Bottom 0.152: Q32.1 18.91,51.37 19.81,52.27 19.81,60.05 v24.23,64.47
N$66  (via drill 0.3)
  Top 0.152: 35.93,59.59 U3.21 36.9,59.57 38.1,58.37 38.1,57.76 v38.71,57.15
  Bottom 0.152: Q54.1 35.82,24.7 38.86,27.74 38.86,57 v38.71,57.15
N$67  (via drill 0.3)
  Top 0.152: U3.22 36.86,60.22 38.41,58.67 38.41,58.52 v38.71,58.22
  Bottom 0.152: Q58.1 36.28,28.51 38.56,30.79 38.56,56.39 38.1,56.84 38.1,57.61 v38.71,58.22
N$68  (via drill 0.3)
  Top 0.152: U3.23 36,60.96 37.03,60.96 v38.71,59.28
  Bottom 0.152: Q59.1 36.28,32.32 38.25,34.29 38.25,56.24 37.8,56.69 37.8,58.37 v38.71,59.28
N$69  (via drill 0.3)
  Top 0.152: U3.24 35.96,61.57 37.49,61.57 v38.71,60.35
  Bottom 0.152: Q60.1 36.28,36.13 37.95,37.8 37.95,56.08 37.49,56.54 37.49,59.13 v38.71,60.35
N$70
  Bottom 0.152: R49.2 17.38,22.8 17.21,22.8
  Bottom 0.254: Q22.2 17.21,22.8
N$71  (via drill 0.3)
  Top 0.152: U3.25 37.96,62.17 v38.71,61.42
  Bottom 0.152: Q61.1 36.42,39.93 37.64,41.15 37.64,55.93 37.19,56.39 37.19,59.89 v38.71,61.42
N$72  (via drill 0.3)
  Top 0.152: U2.18 18.25,57.62 15.11,54.48 13.08,54.48 12.19,55.37 12.19,58.43 12.7,58.94 13.75,58.94 U2.9
  Top 0.406: v15.39,59.44 14.88,58.92 U2.9
  Bottom 0.406: R55.2 C1.1 13.52,58.94 14.02,59.44 v15.39,59.44
N$73  (via drill 0.3)
  Top 0.152: 28.69,58.94 U3.9 | U3.9 30.11,58.92 v30.18,58.98 | U3.9 28.58,58.79 27.43,58.79 27.43,55.32 28.5,54.25 29.41,54.25 30.83,55.67 U3.15 35.95,55.63 37.21,55.63 37.47,55.88 37.47,57.28 37.12,57.62 U3.18
  Bottom 0.152: v30.18,58.98 27.62,58.98 | 27.62,58.98 C2.1 | 27.62,58.98 27.62,60.98 R56.2
N$74  (via drill 0.3)
  Top 0.152: v49.07,59.28 48.71,58.92 U4.9 47.52,58.83 46.63,58.83 46.48,58.67 46.48,55.32 46.94,54.86 v49.68,54.86 | v52.43,56.24 52.51,56.32 U4.16 54.86,56.26 56.13,56.26 56.52,56.64 56.52,57.28 56.17,57.62 U4.18
  Bottom 0.152: v49.07,59.28 46.67,59.28 C3.1 46.15,58.76 R57.2 | v52.43,56.24 51.05,56.24 v49.68,54.86
N$75  (via drill 0.3)
  Top 0.152: U3.26 35.94,62.79 38.41,62.79 v38.71,62.48
  Bottom 0.152: Q62.1 36.13,43.75 37.34,44.96 37.34,55.78 36.88,56.24 36.88,60.66 v38.71,62.48
N$76
  Bottom 0.152: Q96.2 51.64,49.95 R37.2
N$77
  Bottom 0.152: Q19.3 9.45,23.16 10.67,21.95 14.02,21.95 18.44,17.53 18.44,13.26 16.46,11.28 15.02,11.28 V1.BR
N$78
  Top 0.152: Q33.3 36.88,28.96 36.88,24.08 39.78,21.18 44.2,21.18 44.5,20.88 54.12,20.88 V4.TL
N$79
  Bottom 0.152: Q20.3 8.08,33.81 8.08,22.71 9.75,21.03 13.11,21.03 14.92,19.21 V1.TOP
N$80
  Top 0.152: Q36.3 37.19,32.47 37.19,24.23 39.93,21.49 44.35,21.49 44.65,21.18 54.41,21.18 55.63,19.96 57.45,19.96 57.99,19.43 V4.MID
N$81
  Top 0.152: Q37.3 37.49,35.97 37.49,24.38 40.08,21.79 44.5,21.79 44.81,21.49 54.71,21.49 55.78,20.42 58.83,20.42 60.45,18.8 V4.TOP
N$82
  Top 0.152: Q39.3 37.8,39.48 37.8,24.54 40.23,22.1 44.65,22.1 44.96,21.79 54.86,21.79 55.93,20.73 59.59,20.73 60.5,19.81 61.11,19.81 62.23,18.69 V4.TR
N$83
  Top 0.152: Q40.3 38.1,42.98 38.1,24.69 40.39,22.4 44.81,22.4 45.11,22.1 55.02,22.1 56.08,21.03 59.74,21.03 60.66,20.12 61.42,20.12 63.86,17.68 63.86,13.87 62.75,12.76 V4.DOT
N$84
  Top 0.152: Q41.3 38.41,46.49 38.41,24.84 40.54,22.71 44.96,22.71 45.26,22.4 55.17,22.4 56.24,21.34 59.89,21.34 60.81,20.42 61.57,20.42 64.16,17.83 64.16,12.5 62.84,11.18 V4.BR
N$85
  Top 0.254: Q38.3 33.05,22.12 Q35.1
N$86
  Top 0.254: Q42.3 33.05,25.93 Q34.1
N$87
  Top 0.254: Q43.3 33.05,29.74 Q33.1
N$88
  Top 0.152: Q80.2 44.3,49.83 R45.2
N$89
  Top 0.254: Q44.3 33.05,33.55 Q36.1
N$90
  Top 0.254: Q45.3 33.05,37.36 Q37.1
N$91
  Top 0.254: Q46.3 33.05,41.17 Q39.1
N$92
  Top 0.254: Q47.3 33.05,44.98 Q40.1
N$93
  Top 0.254: Q48.3 33.05,48.79 Q41.1
N$94  (via drill 0.3)
  Top 0.152: U3.27 38.63,63.47 v38.71,63.55
  Bottom 0.152: Q63.1 32.43,47.4 36.73,47.4 37.03,47.7 37.03,55.63 36.58,56.08 36.58,61.42 v38.71,63.55
N$95
  Top 0.152: R18.2 30.12,28.73 Q43.2
N$96
  Top 0.152: R19.2 30.13,32.66 Q44.2
N$97
  Top 0.152: R20.2 30.12,36.35 Q45.2
N$98
  Top 0.152: R21.2 30.13,40.28 Q46.2
N$99
  Top 0.152: R22.2 30,44.22
  Top 0.254: 30,44.22 Q47.2
N$100
  Top 0.152: R17.2 29.88,25.3
  Top 0.254: 29.88,25.3 Q42.2
N$101  (via drill 0.3)
  Top 0.152: U3.28 38.21,64.12 v38.71,64.62
  Bottom 0.152: Q64.1 35.67,51.37 36.73,52.43 36.73,55.47 36.27,55.93 36.27,62.18 v38.71,64.62
N$102
  Top 0.152: Q38.1 29.81,23.07 28.5,24.38 24.84,24.38 23.77,25.45 23.77,52.27 24.99,53.49 24.99,61.72 27.43,64.16 28.67,64.16 U3.1
N$103
  Top 0.152: Q42.1 25.09,26.88 24.08,27.89 24.08,52.12 25.3,53.34 25.3,61.42 27.28,63.4 28.64,63.4 U3.2
N$104
  Top 0.152: Q43.1 25.54,30.69 24.38,31.85 24.38,51.97 25.6,53.19 25.6,60.96 27.43,62.79 28.68,62.79 U3.3
N$105
  Top 0.152: Q44.1 25.54,34.5 24.69,35.36 24.69,51.82 25.91,53.03 25.91,60.5 27.58,62.18 28.7,62.18 U3.4
N$106
  Top 0.152: Q45.1 25.85,38.31 24.99,39.17 24.99,51.66 26.21,52.88 26.21,60.05 27.58,61.42 28.61,61.42 U3.5
N$107
  Top 0.152: U3.6 27.64,60.87 26.52,59.74 26.52,52.73 25.3,51.51 25.3,43.43 26.52,42.22 30.1,42.22 Q46.1
N$108
  Top 0.152: Q47.1 26.61,45.93 25.6,46.94 25.6,51.36 26.82,52.58 26.82,59.28 27.74,60.2 28.69,60.2 U3.7
N$109
  Top 0.152: U3.8 28.69,59.59 27.74,59.59 27.13,58.98 27.13,52.81 Q48.1
N$110  (via drill 0.3)
  Top 0.152: U4.21 56.1,59.57 56.69,58.98 56.69,57.91 v57.61,57
  Bottom 0.152: Q86.1 55.13,25.56 56.39,26.21 56.39,55.78 v57.61,57
N$111
  Top 0.152: 30.16,21.21 Q38.2 30.19,21.32 29.72,21.79 28.48,21.79 R16.2
N$112
  Top 0.152: Q34.3 36.1,24.4 39.62,20.88 44.04,20.88 44.35,20.57 51.24,20.57 V4.BL
N$113
  Top 0.152: U5.1 16.75,68.89 15.54,68.89 15.09,68.43 15.09,67.36 14.75,67.02 C7.1
N$114  (via drill 0.3)
  Top 0.152: U4.22 56.06,60.22 57,59.28 57,58.67 v57.61,58.06
  Bottom 0.152: Q90.1 54.52,29.37 56.08,30.33 56.08,56.54 v57.61,58.06
N$115  (via drill 0.3)
  Top 0.152: U4.23 55.87,60.87 v57.61,59.13
  Bottom 0.152: Q91.1 53.91,33.18 55.78,34.44 55.78,57.3 v57.61,59.13
N$116  (via drill 0.3)
  Top 0.152: U4.24 56.29,61.52 v57.61,60.2
  Bottom 0.152: Q92.1 53.93,36.87 55.47,37.8 55.47,58.06 v57.61,60.2
N$117  (via drill 0.3)
  Top 0.152: U4.25 56.68,62.17 v57.61,61.27
  Bottom 0.152: Q93.1 53.48,40.68 55.17,42.37 55.17,58.83 v57.61,61.27
N$118  (via drill 0.3)
  Top 0.152: U4.26 57.27,62.82 v57.61,62.33
  Bottom 0.152: Q94.1 54.24,44.49 54.86,45.11 54.86,59.59 v57.61,62.33
N$119  (via drill 0.3)
  Top 0.152: V3.TR 45.94,16.15 39.17,16.15 37.19,18.14 37.19,18.9 v37.8,19.51
  Bottom 0.152: Q49.3 25.3,30.31 25.3,23.01 26.82,21.49 34.9,21.49 36.88,19.51 v37.8,19.51
N$120  (via drill 0.3)
  Top 0.152: v38.86,19.51 39.17,19.81 42.37,19.81 42.75,19.43 V3.MID
  Bottom 0.152: Q53.3 24.69,37.32 24.69,22.71 26.52,20.88 34.29,20.88 37.34,17.83 38.1,17.83 38.86,18.59 v38.86,19.51
N$121  (via drill 0.3)
  Top 0.152: U4.27 57.52,63.47 v57.61,63.4
  Bottom 0.152: Q95.1 54.11,48.17 54.56,48.62 54.56,60.35 v57.61,63.4
N$122
  Bottom 0.152: Q55.3 24.38,40.83 24.38,22.55 26.36,20.57 34.14,20.57 37.19,17.53 38.25,17.53 39.47,18.75 40.91,18.75 V3.TL
N$123
  Bottom 0.152: Q56.3 24.08,44.33 24.08,22.4 26.67,19.81 26.67,19.66 26.98,19.36 26.98,18.44 27.74,17.68 30.63,17.68 31.24,18.29 35.97,18.29 37.05,17.21 V3.BL
N$124
  Bottom 0.152: Q57.3 23.77,47.84 23.77,22.25 26.36,19.66 26.36,19.51 26.67,19.2 26.67,18.29 28.8,16.15 37.64,16.15 38.73,15.06 V3.BOT
N$125
  Bottom 0.254: Q54.3 29.41,23.75 Q51.1
N$126
  Bottom 0.254: Q58.3 29.41,27.56 Q50.1
N$127
  Bottom 0.254: Q59.3 29.41,31.37 Q49.1
N$128
  Bottom 0.254: Q60.3 29.41,35.18 Q52.1
N$129
  Bottom 0.254: Q61.3 29.41,38.99 Q53.1
N$130
  Bottom 0.254: Q62.3 29.41,42.8 Q55.1
N$131
  Bottom 0.254: Q63.3 29.41,46.61 Q56.1
N$132
  Bottom 0.254: Q64.3 29.41,50.42 Q57.1
N$133  (via drill 0.3)
  Top 0.152: U4.28 54.92,64.01 57.91,64.01 58.52,63.4 v58.52,62.33
  Bottom 0.152: Q96.1 52.5,54.25 53.34,54.25 54.25,55.17 54.25,60.5 56.84,63.09 56.84,64.01 57.91,64.01 58.52,63.4 v58.52,62.33
N$134
  Bottom 0.152: Q59.2 32.33,30.48 R25.2
N$135
  Bottom 0.152: R26.2 34.04,34.23 Q60.2
N$136
  Bottom 0.152: R27.2 34.17,38.04 Q61.2
N$137
  Bottom 0.152: Q62.2 32.45,42.04 R28.2
N$138
  Bottom 0.152: R29.2 34.17,45.66 Q63.2
N$139
  Bottom 0.152: Q58.2 32.45,26.8 R24.2
N$140
  Top 0.152: Q70.1 42.61,25.05 39.62,28.04 39.62,52.43 44.04,56.84 44.04,61.42 46.63,64.01 47.5,64.01 U4.1
N$141
  Bottom 0.406: V5.FIL_P 71.44,9.12 R53.1
N$142  (via drill 0.3)
  Top 0.152: U1.14 88.47,36.8 86.56,38.71 86.56,43.13 85.87,43.83 C12.1 v85.65,47.7 | v87.17,23.47 93.73,23.47 96.16,25.91 v96.16,45.57
  Bottom 0.152: v85.65,47.7 85.65,46.95 B1.+1 95.87,45.27 v96.16,45.57 | B1.+2 84.14,23.47 v87.17,23.47
N$143
  Bottom 0.406: V3.FIL_P 40.96,9.12 R48.1
N$144
  Bottom 0.406: V1.FIL_P 10.48,9.12 R46.1
N$145
  Top 0.152: R62.1 R63.2 | C8.1 6.81,67.27 R62.1 | R62.1 11.49,65.53 15.09,65.53 16.73,67.17 U5.3
N$146  (via drill 0.3)
  Top 0.152: R58.2 37.34,74.52 36.73,75.13 31.92,75.13 R59.1 30.87,74.52 v29.26,74.52
  Bottom 0.152: R100.2 29.28,74.54 v29.26,74.52
N$147
  Top 0.152: R61.2 R58.1 37.4,72.54 41.6,72.54 42.1,72.05 U6.3
N$148
  Top 0.152: U5.4 20.37,66.14 25.91,66.14 27.43,67.67 R64.1 25.63,69.83 C10.1
N$149
  Bottom 0.152: U7.9 64.9,35.66 X3.P$2 C17.1
N$150
  Bottom 0.152: R43.2 34.17,22.8 Q54.2
N$151
  Bottom 0.406: V4.FIL_P 56.2,9.12 R52.1
N$152
  Bottom 0.406: V6.FIL_P 86.68,9.12 R54.1
N$153
  Bottom 0.152: U7.10 X3.P$1 C18.1
N$154  (via drill 0.3)
  Top 0.152: v49.23,64.47 49.68,64.01 50.14,64.01 51.51,62.64 51.51,55.47 53.65,53.34 C20.2
  Bottom 0.152: U8.2 47.59,64.77 49.07,64.77 49.23,64.62 v49.23,64.47
N$155
  Bottom 0.152: U8.15 54.73,72.54 55.78,72.54 55.93,72.39 55.93,69.65 59.44,66.14 59.44,65.53 61.27,63.7 64.01,63.7 66.14,65.84 X2.3
N$156  (via drill 0.3)
  Top 0.152: v37.8,21.34 36.58,20.12 36.58,15.54 38.1,14.02 42.37,14.02 45.21,11.18 V3.BR
  Bottom 0.152: Q51.3 26.36,22.86 27.13,22.1 35.36,22.1 36.12,21.34 v37.8,21.34
N$157  (via drill 0.3)
  Top 0.152: V3.TOP 44.28,17.68 40.39,17.68 39.78,18.29 38.1,18.29 v37.8,18.59
  Bottom 0.152: Q52.3 24.99,33.81 24.99,22.86 26.67,21.18 34.59,21.18 37.19,18.59 v37.8,18.59
N$158  (via drill 0.3)
  Top 0.152: v37.8,20.42 37.34,20.42 36.88,19.96 36.88,17.98 39.01,15.85 44.81,15.85 46.99,13.66 V3.DOT
  Bottom 0.152: Q50.3 25.6,26.8 25.6,23.16 26.98,21.79 35.2,21.79 36.58,20.42 v37.8,20.42
N$159
  Top 0.152: Q67.3 52.13,23.92 53.34,22.71 55.32,22.71 56.39,21.64 60.05,21.64 60.96,20.73 61.72,20.73 68.58,13.87 83.34,13.87 V6.BOT
N$160
  Bottom 0.152: X2.2 65.23,68.35 65.23,65.38 63.86,64.01 61.42,64.01 59.74,65.68 59.74,66.29 56.24,69.8 56.24,72.69 55.78,73.15 53.65,73.15 53.19,72.69 53.19,72.24 53.47,71.96 U8.16
N$161
  Top 0.152: Q65.3 53.34,30.51 53.34,25.15 55.17,23.32 55.63,23.32 56.69,22.25 60.35,22.25 61.27,21.34 62.03,21.34 65.08,18.29 70.26,18.29 71.02,17.53 76.05,17.53 77.57,19.05 86.42,19.05 V6.TL
N$162
  Top 0.152: Q68.3 53.65,34.02 53.65,25.3 55.32,23.62 55.78,23.62 56.84,22.55 60.5,22.55 61.42,21.64 62.18,21.64 64.01,19.81 71.93,19.81 72.24,19.51 72.24,19.2 72.39,19.05 72.39,18.9 73.15,18.14 74.37,18.14 74.98,18.75 74.98,19.2 75.59,19.81 88.52,19.81 V6.MID
N$163
  Top 0.152: Q69.3 53.95,37.52 53.95,25.45 55.47,23.93 55.93,23.93 57,22.86 60.66,22.86 61.57,21.95 62.33,21.95 64.16,20.12 72.39,20.12 72.69,19.81 72.69,19.2 72.85,19.05 72.85,18.9 73.3,18.44 74.22,18.44 74.52,18.75 74.52,19.05 74.68,19.2 74.68,19.51 75.29,20.12 88.24,20.12 88.54,20.42 89.5,20.42 V6.TOP
N$164
  Top 0.152: Q71.3 54.25,41.03 54.25,25.6 55.63,24.23 56.08,24.23 57.15,23.16 60.81,23.16 61.72,22.25 62.48,22.25 64.31,20.42 88.09,20.42 88.39,20.73 90.68,20.73 92.81,18.59 92.81,17.31 V6.TR
N$165
  Top 0.152: Q72.3 54.56,44.53 54.56,25.76 55.78,24.54 56.24,24.54 57.3,23.47 60.96,23.47 61.87,22.55 62.64,22.55 64.47,20.73 74.68,20.73 75.29,20.73 87.94,20.73 88.24,21.03 90.83,21.03 94.34,17.53 94.34,13.72 93.42,12.8 92.75,12.8 V6.DOT
N$166
  Top 0.152: V6.BR 91.17,11.12 92.51,11.12 94.64,13.26 94.64,17.68 90.98,21.34 88.09,21.34 87.78,21.03 68.12,21.03 65.23,23.93 63.25,23.93 63.09,23.77 57.45,23.77 56.39,24.84 55.93,24.84 54.86,25.91 54.86,47.09 52.13,49.83 Q73.3
N$167
  Top 0.254: Q70.3 49.27,25.05 Q67.1
N$168
  Top 0.254: Q74.3 49.27,28.86 Q66.1
N$169
  Top 0.254: Q75.3 49.27,32.67 Q65.1
N$170
  Top 0.254: Q76.3 49.27,36.48 Q68.1
N$171
  Top 0.254: Q77.3 49.27,40.3 Q69.1
N$172
  Top 0.254: Q78.3 49.27,44.1 Q71.1
N$173
  Top 0.254: Q79.3 49.27,47.91 Q72.1
N$174
  Top 0.254: Q80.3 49.27,51.73 Q73.1
N$175  (via drill 0.3)
  Top 0.152: RX.1 72.69,70.41 65.68,63.4 v64.77,63.4
  Bottom 0.152: U8.23 54.71,67.36 57.15,67.36 61.11,63.4 v64.77,63.4
N$176
  Top 0.152: Q75.2 44.45,30.77 R39.2
N$177
  Top 0.152: Q76.2 44.57,34.59 R40.2
N$178
  Top 0.152: Q77.2 44.45,38.4 R41.2
N$179
  Top 0.152: Q78.2 44.57,42.2 R42.2
N$180
  Top 0.152: Q79.2 44.33,46.02 R44.2
N$181
  Top 0.152: Q74.2 44.32,26.96 R38.2
N$182
  Top 0.152: Q74.1 41.54,28.86 39.93,30.48 39.93,52.27 44.35,56.69 44.35,61.11 46.63,63.4 47.54,63.4 U4.2
N$183
  Top 0.152: Q75.1 41.85,32.67 40.23,34.29 40.23,52.12 44.65,56.54 44.65,60.81 46.63,62.79 47.58,62.79 U4.3
N$184
  Top 0.152: Q76.1 41.85,36.48 40.54,37.8 40.54,51.97 44.96,56.39 44.96,60.35 46.79,62.18 47.59,62.18 U4.4
N$185
  Top 0.152: Q77.1 42.61,40.3 40.84,42.06 40.84,51.82 45.26,56.24 45.26,60.05 46.63,61.42 47.51,61.42 U4.5
N$186
  Top 0.152: Q78.1 42.15,44.1 41.15,45.11 41.15,51.66 45.57,56.08 45.57,59.74 46.63,60.81 47.55,60.81 U4.6
N$187
  Top 0.152: Q79.1 42.31,47.91 41.45,48.77 41.45,51.51 45.87,55.93 45.87,59.44 46.63,60.2 47.59,60.2 U4.7
N$188
  Top 0.152: U4.8 47.59,59.59 46.63,59.59 46.18,59.13 46.18,51.77 Q80.1
  Top 0.254: 46.22,51.66 Q80.1
N$189  (via drill 0.3)
  Top 0.152: TX.1 56.84,71.48 56.69,71.63 56.69,73 55.93,73.76 52.88,73.76 51.05,71.93 51.05,68.73 51.66,68.12 v52.58,68.12
  Bottom 0.152: v52.58,68.12 54.6,68.12 U8.22
N$190
  Top 0.152: C14.1 72.43,37.55 U7.21
N$191
  Top 0.152: CR2.1 CR1.2
N$192
  Top 0.152: Q70.2 44.32,23.16 R51.2
N$193
  Top 0.152: Q66.3 53.03,27.01 53.03,24.99 55.02,23.01 55.47,23.01 56.54,21.95 60.2,21.95 61.11,21.03 61.87,21.03 66.9,16 83.88,16 V6.BL
N$194
  Top 0.152: PWR.1 79.39,69.81 R70.1
N$195
  Top 0.152: RX.2 72.86,74.05 R68.2
N$196
  Top 0.152: R69.2 59.3,74.05 TX.2
N$197
  Top 0.152: CR3.1 CR2.2
N$198
  Top 0.152: CR4.1 CR3.2
N$199
  Top 0.152: R66.2 62.23,51.51 U7.2
  Bottom 0.152: U7.2 64.21,53.49 64.62,53.49 70.1,58.98 94.89,58.98 JP1.2
N$200
  Bottom 0.152: Q81.3 42.37,31.27 42.37,23.47 44.81,21.03 76.2,21.03 77.47,19.76 V5.TR
N$201
  Bottom 0.152: Q85.3 41.76,38.03 41.76,23.16 44.5,20.42 72.85,20.42 73.66,19.61 V5.MID 73.53,19.43
N$202
  Bottom 0.152: Q87.3 41.45,41.66 41.45,23.01 44.35,20.12 56.84,20.12 57.45,19.51 57.45,18.75 57.76,18.44 59.13,18.44 59.44,18.75 59.44,19.51 60.05,20.12 69.8,20.12 71.12,18.8 V5.TL 71.44,18.94
N$203
  Bottom 0.152: Q88.3 41.15,45.17 41.15,22.86 42.22,21.79 42.22,19.2 42.37,19.05 42.37,18.9 42.82,18.44 43.89,18.44 44.35,18.9 44.35,19.36 44.81,19.81 53.34,19.81 55.78,17.37 60.81,17.37 61.87,18.44 68.73,18.44 69.85,17.32 V5.BL
N$204
  Bottom 0.152: Q89.3 40.84,48.55 40.84,22.71 41.91,21.64 41.91,19.05 42.06,18.9 42.06,18.75 44.65,16.15 57.3,16.15 59.89,16.15 68.05,16.15 V5.BOT
N$205
  Bottom 0.254: Q86.3 46.19,25.69 Q83.1
N$206
  Bottom 0.254: Q90.3 46.06,29.63 Q82.1
N$207
  Bottom 0.254: Q91.3 46.19,33.31 Q81.1
N$208
  Bottom 0.254: Q92.3 46.19,36.99 Q84.1
N$209
  Bottom 0.254: Q93.3 46.31,40.68 Q85.1
N$210
  Bottom 0.254: Q94.3 46.31,44.61 Q87.1
N$211
  Bottom 0.254: Q95.3 46.19,48.42 Q88.1
N$212
  Bottom 0.254: Q96.3 46.19,52.11 Q89.1
N$213
  Top 0.152: CR5.1 CR4.2
N$214
  Bottom 0.152: Q91.2 51.39,31.28 R32.2
N$215
  Bottom 0.152: Q92.2 51.39,34.97 R33.2
N$216
  Bottom 0.152: 49.43,38.71 51.4,38.71 R34.2
  Bottom 0.254: Q93.2 49.43,38.71
N$217
  Bottom 0.152: 49.55,42.52 51.68,42.52 R35.2
  Bottom 0.254: Q94.2 49.55,42.52
N$218
  Bottom 0.152: 49.55,46.33 R36.2
  Bottom 0.254: Q95.2 49.55,46.33
N$219
  Bottom 0.152: 49.55,27.66 R31.2
  Bottom 0.254: Q90.2 49.55,27.66
N$220
  Top 0.152: R67.2 62.79,49.53 U7.3
  Bottom 0.152: U7.3 70.87,57.61 93.27,57.61 93.73,58.06 96.62,58.06 97.23,58.67 97.23,60.05 95.86,61.42 95.71,61.42 JP1.1
N$221
  Top 0.152: TX6.1 CR5.2
N$222
  Top 0.152: R73.2 TX6.2
N$223  (via drill 0.3)
  Top 0.152: CR1.1 90.68,8.84 94.94,13.11 94.94,19.05 94.18,19.81 v94.03,19.81 | Q97.3 v92.66,24.38
  Bottom 0.152: v92.66,24.38 92.66,21.18 v94.03,19.81
N$224
  Top 0.152: Q97.1 79.74,25.3 R75.2
N$225
  Top 0.152: P1.P$2 77.57,47.9 | 77.57,47.9 76.59,47.9 R76.2 | 77.57,47.9 77.72,47.75 77.72,43.43 75.89,41.6 75.47,41.6 Q98.3
N$226
  Top 0.152: Q98.1 76.39,45.67 R77.2
N$228  (via drill 0.3)
  Top 0.203: C21.1 53.09,71.37 v52.32,72.14
  Bottom 0.203: U8.17 54.66,71.37 53.09,71.37 v52.32,72.14
N$231
  Bottom 0.152: 49.42,23.72 51.32,23.72 R50.2
  Bottom 0.254: Q86.2 49.42,23.72
N$238
  Bottom 0.152: Q83.3 43.45,23.45 45.26,21.64 76.5,21.64 80.31,17.83 80.31,13.11 78.38,11.18 V5.BR
N$239
  Bottom 0.152: Q84.3 42.06,34.65 42.06,23.32 44.65,20.73 75.44,20.73 75.88,20.28 V5.TOP
N$240
  Bottom 0.152: Q82.3 42.67,27.9 42.67,23.62 44.96,21.34 76.35,21.34 80.01,17.68 80.01,14.17 78.64,12.8 77.51,12.8 V5.DOT
PLATE  (via drill 0.3)  (1 unrouted)
  Top 0.152: C5.1 30.33,71.48 v29.57,72.24 | V6.GRID_P 88.9,7.37 88.85,7.32 | 27.94,7.42 28.04,7.32 | V3.GRID_P 43.18,7.42 43.28,7.32 | V4.GRID_P 58.42,7.42 58.52,7.32 | V5.GRID_P 73.66,7.37 73.61,7.32 | 12.7,7.42 12.5,7.62 7.62,7.62 6.72,8.52 R73.1
  Top 0.381: 18.59,20.83 18.59,17.98 18.9,17.68 18.9,13.11 15.85,10.06 13.18,10.06 V1.GRID_P 12.7,7.42 12.8,7.32 13.41,7.32 | 27.94,7.42 V2.GRID_P 28.42,10.06 32.77,10.06 35.05,12.34 35.05,21.18 35.04,21.17 Q35.2 | 51.05,49.83 51.05,52.88 v47.55,52.88 | Q73.2 50.91,49.83 51.05,49.68
  Top 0.406: Q9.2 19.81,47.69 19.81,43.88 | 19.81,43.88 19.81,40.07 | 19.81,40.07 19.81,36.26 | 19.81,36.26 19.81,32.45 | 19.81,32.45 19.81,28.64 | 19.81,28.64 19.81,24.83 | 19.81,24.83 19.81,21.03 Q4.2 18.59,20.83 | Q3.2 19.81,24.83 | Q2.2 19.81,28.64 | Q5.2 19.81,32.45 | Q6.2 19.81,36.26 | Q1.2 19.81,40.07 | Q7.2 19.81,43.88 | Q41.2 35.05,47.84 35.05,44.04 | 35.05,44.04 35.05,40.23 | 35.05,40.23 35.05,36.27 | 35.05,36.27 35.05,32.61 | 35.05,32.61 35.05,28.8 | 35.05,28.8 35.05,24.99 | 35.05,24.99 35.05,21.18 | 34,21.18 Q35.2 | Q34.2 35.04,24.98 35.05,24.99 | Q33.2 35.04,28.79 35.05,28.8 | Q36.2 35.04,32.6 35.05,32.61 | Q37.2 34.91,36.41 35.05,36.27 | Q39.2 35.04,40.22 35.05,40.23 | Q40.2 35.04,44.03 35.05,44.04 | Q72.2 51.04,46.02 51.05,46.02 | 51.05,49.83 51.05,49.68 51.05,46.02 | 51.05,46.02 51.05,42.22 | 51.05,42.22 51.05,38.41 | 51.05,38.41 51.05,34.75 | 51.05,34.75 51.05,30.94 | 51.05,30.94 51.05,26.98 | 51.05,26.98 51.05,23.32 50.19,23.32 Q67.2 | Q66.2 51.04,26.96 51.05,26.98 | Q65.2 50.89,30.77 51.05,30.94 | Q68.2 50.89,34.59 51.05,34.75 | Q69.2 51.04,38.4 51.05,38.41 | Q71.2 51.04,42.2 51.05,42.22 | 88.85,7.32 73.61,7.32 58.52,7.32 43.28,7.32 28.04,7.32 13.41,7.32
  Bottom 0.152: v29.57,72.24 29.57,71.93
  Bottom 0.254: 27.43,22.86 28.46,22.86
  Bottom 0.381: 13.56,22.71 13.87,22.71 18.9,17.68 18.9,13.11 15.7,9.91 13.34,9.91 V1.GRID_P | 23.32,21.95 23.32,19.66 27.89,15.09 27.89,10.59 V2.GRID_P | v47.55,52.88 44.65,52.88 44.5,52.73
  Bottom 0.406: 27.13,51.21 27.43,50.9 27.43,49.53 | 27.13,51.21 25.45,51.21 23.32,49.07 23.32,21.95 | 44.5,50.21 Q89.2 44.57,50.21 44.5,50.14 | 44.5,50.21 44.5,50.14 | 44.5,50.14 44.5,46.52 | 44.5,46.52 44.5,42.71 | 44.5,42.71 44.5,38.78 | 44.5,38.78 44.5,35.09 | 44.5,35.09 44.5,31.41 | 44.5,31.41 44.5,27.73 | 44.5,27.73 44.5,23.77 45.55,23.77 Q83.2 | Q82.2 44.5,27.73 | Q81.2 44.5,31.41 | Q84.2 44.5,35.09 | Q85.2 44.5,38.78 | Q87.2 44.5,42.71 | Q88.2 44.5,46.52 | 27.43,49.53 27.43,45.57 | 27.43,45.57 27.43,41.91 | 27.43,41.91 27.43,38.1 | 27.43,38.1 27.43,34.14 | 27.43,34.14 27.43,30.33 | 27.43,30.33 27.43,26.67 | 27.43,26.67 27.43,22.8 Q51.2 | Q50.2 28.46,26.67 27.43,26.67 | Q49.2 28.46,30.33 27.43,30.33 | Q52.2 28.46,34.14 27.43,34.14 | Q53.2 28.46,38.1 27.43,38.1 | Q55.2 28.46,41.91 27.43,41.91 | Q56.2 28.46,45.57 27.43,45.57 | Q57.2 28.46,49.53 27.43,49.53 | Q25.2 11.54,49.53 10.52,49.53 10.52,45.57 | 10.52,45.57 10.52,41.91 | 10.52,41.91 10.52,38.1 | 10.52,38.1 10.52,34.29 | 10.52,34.29 10.52,30.48 | 10.52,30.48 10.52,26.52 | 10.52,26.52 10.52,22.8 Q19.2 11.54,22.71 13.56,22.71 | Q18.2 11.54,26.52 10.52,26.52 | Q17.2 11.54,30.48 10.52,30.48 | Q20.2 11.54,34.29 10.52,34.29 | Q21.2 11.54,38.1 10.52,38.1 | Q23.2 11.54,41.91 10.52,41.91 | Q24.2 11.54,45.57 10.52,45.57 | 27.13,51.21 27.13,52.27 32.46,57.61 32.46,63.4 31.24,64.62 31.24,65.08 | 31.24,65.08 31.24,69.34 | 31.24,69.34 31.24,70.56 v29.57,72.24 | 44.5,50.21 44.5,52.73 44.5,53.49 43.28,54.71 42.98,54.71 41.15,56.54 41.15,63.25 39.01,65.38 31.55,65.38 31.24,65.08 | R100.1 31.24,69.34 | 31.24,69.34
  pour Top: 38.25,71.63 33.53,71.63 33.53,73.3 28.65,73.3 28.65,69.49 38.25,69.49
RESET  (via drill 0.3)
  Top 0.152: v65.08,60.81 65.08,58.22 64.16,57.3 U7.1 61.52,53.34 C20.1 | v66.75,61.87 78.79,61.87 80.06,60.6 S1.3
  Bottom 0.152: R65.1 81.05,61.61 S1.3 | v65.08,60.81 66.14,61.87 v66.75,61.87
RX  (via drill 0.3)  (1 unrouted)
  Top 0.152: v49.23,63.55 50.14,63.55 51.21,62.48 51.21,61.42 51.05,61.27 51.05,55.32 54.73,51.65
  Bottom 0.152: U8.1 48.46,64.16 49.07,63.55 v49.23,63.55
SCL  (via drill 0.3)
  Top 0.152: U2.12 16.43,56.97 17.53,58.06 17.53,63.7 19.36,65.53 28.19,65.53 | 28.19,65.53 49.84,65.53 | U3.12 30.45,56.97 30.79,57.3 30.79,59.44 29.87,60.35 29.87,64.01 v30.33,64.47 | v28.19,66.14 28.19,65.53 | U4.12 49.35,56.97 49.84,57.45 v49.84,62.79 | v49.84,66.29 49.84,65.53 | 49.84,65.53 58.37,65.53 62.03,61.87 65.84,61.87 67.67,60.05 67.67,58.67 70.36,55.98 U7.28 | 90.19,41.95 R71.1 | U1.16 90.07,39.47 R71.1 | U7.28 80.42,55.98 86.87,49.53 86.87,46.79 89.15,44.5 89.15,42.99 R71.1 | 71.98,55.98 U7.28
  Bottom 0.152: v30.33,64.47 v28.19,66.14 | v49.84,62.79 v49.84,66.29
SDA  (via drill 0.3)
  Top 0.152: U2.13 16.39,56.32 17.98,57.91 17.98,63.55 19.66,65.23 30.94,65.23 | 30.94,65.23 50.6,65.23 | 50.6,65.23 58.22,65.23 61.87,61.57 65.68,61.57 67.36,59.89 67.36,58.52 70.1,55.78 70.1,55.02 71.68,53.44 U7.27 82.5,53.44 86.56,49.38 86.56,44.2 | U3.13 30.71,56.32 31.09,56.69 31.09,59.59 30.18,60.5 30.18,63.4 30.94,64.16 30.94,65.23 | U4.13 49.16,56.32 50.6,57.76 v50.6,62.03 | v50.6,64.62 50.6,65.23 | U1.15 90.17,38.1 88.7,38.1 86.87,39.93 86.87,43.43 86.56,43.74 86.56,44.2 | R72.1 87.46,44.2 86.56,44.2
  Bottom 0.152: v50.6,62.03 v50.6,64.62
SW1
  Top 0.152: U7.11 70.81,23.93 72.85,23.93 74.52,22.25 87.17,22.25 87.48,22.55 93.88,22.55 96.16,20.27 96.16,12.5 92.05,8.38 92.05,7.32 87.94,3.2 87.94,2.44 87.17,1.68 11.12,1.68 10.4,2.4 SW1.S1 9.06,3.35 R78.2
SW2
  Top 0.152: U7.12 66.45,25.76 66.75,25.76 70.56,21.95 87.33,21.95 87.63,22.25 93.73,22.25 95.86,20.12 95.86,12.65 91.75,8.53 91.75,7.47 87.63,3.35 87.63,2.59 87.02,1.98 26.67,1.98 25.64,3.01 SW2.S1 R79.2
SW3
  Top 0.152: U7.13 64.21,25.45 66.6,25.45 70.41,21.64 87.48,21.64 87.78,21.95 93.57,21.95 95.56,19.96 95.56,12.8 91.44,8.69 91.44,7.62 88.85,5.03 86.41,5.03 85.8,4.42 58.52,4.42 57.15,3.05 57.15,2.74 56.69,2.29 41.6,2.29 40.88,3.01 SW3.S1 R80.2
SW4  (via drill 0.3)
  Top 0.152: v68.12,22.4 69.19,21.34 87.63,21.34 87.94,21.64 93.42,21.64 95.25,19.81 95.25,12.95 91.14,8.84 91.14,7.77 88.7,5.33 86.26,5.33 85.65,4.72 57,4.72 56.12,3.85 SW4.S1 R81.2
  Bottom 0.152: U7.14 64.72,22.4 v68.12,22.4
SW5
  Top 0.152: R82.2 SW5.S1
  Bottom 0.152: U7.15 72.8,21.95 76.66,21.95 83.36,15.24 83.36,14.33 83.67,14.02 85.65,14.02 87.78,11.89 87.78,6.55 85.95,4.72 82.91,4.72 81.53,6.1 79.55,6.1 78.18,4.72 74.68,4.72 73.3,3.35 SW5.S1
SW6
  Top 0.152: R83.2 SW6.S1
  Bottom 0.152: U7.16 75.03,22.25 76.81,22.25 83.06,16 85.65,16 89.92,11.73 89.92,6.86 86.6,3.54 SW6.S1
TEMP
  Top 0.152: U7.26 73.29,50.9 Q99.2
TX  (via drill 0.3)
  Top 0.152: v52.12,64.62 v52.12,57.45 | R67.1 54.1,49.53 52.88,50.75 52.88,52.73 v49.68,55.93
  Bottom 0.152: U8.5 48.92,66.75 49.23,67.06 50.29,67.06 52.12,65.23 v52.12,64.62 | v52.12,57.45 51.21,57.45 v49.68,55.93
  Bottom 0.203: U8.5
VS5
  pour Top: 36.27,69.19 36.27,65.84 40.69,65.84 40.69,72.09 38.56,72.09 38.56,69.19
VSW3
  pour Top: 22.86,71.78 22.86,75.13 17.98,75.13 17.98,69.95 12.65,69.95 12.65,68.28 15.09,68.28 15.09,69.65 18.14,69.65 18.14,68.58 19.81,68.58 19.81,71.78

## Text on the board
tPlace: VFD CLOCK V2
tStop: RUARK / MMXVII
